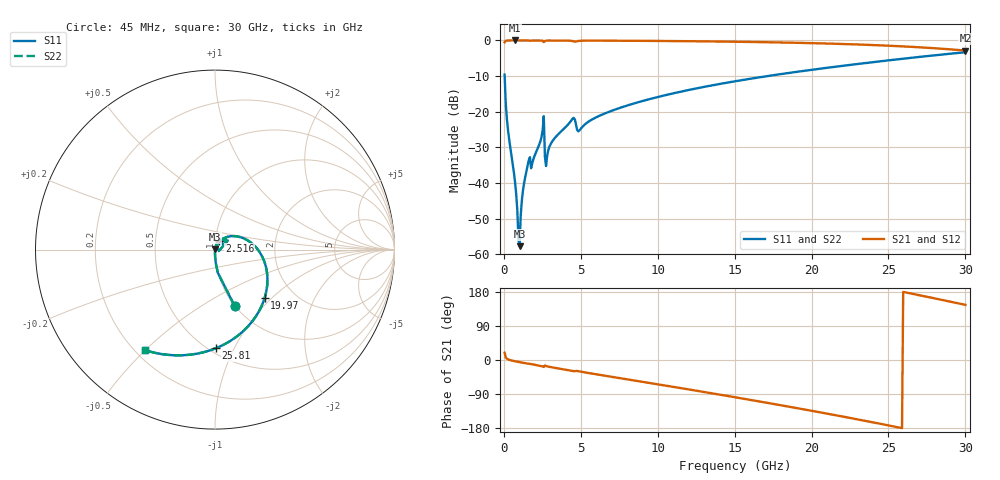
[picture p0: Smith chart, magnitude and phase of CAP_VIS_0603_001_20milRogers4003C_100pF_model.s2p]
! S-parameter model data by Modelithics Inc.  support@modelithics.com  813-866-6335  Tampa FL USA
! S-Parameter data specifications:
! Substrate: 20-mil Rogers 4003C, substrate thickness, H=0.508mm, Dielectric constant, Er=3.75
! PCB Mounting Pad Footprint: Pad width, PadW=0.90mm , Pad length, PadL=1.00mm , Pad gap, PadG (edge-to-edge)=1.00mm , Reference planes=3.0mm apart
! Created Wed Nov 18 13:31:23 2015
# hz S ma R 50
! 2 Port Network Data from SP1.SP block
! freq  magS11  angS11  magS21  angS21  magS12  angS12  magS22  angS22
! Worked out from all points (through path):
!   401 points, 45 MHz to 30 GHz, reference 50 ohm
!   highest |S21| = -0.01 dB at 719 MHz (marker M1); lowest = -2.8 dB at 30 GHz (marker M2)
!   group delay of S21, straight-line fit = 19.8 ps
!   lowest |S11| = -57.7 dB at 1.019 GHz (marker M3), VSWR 1.00, Z = 50.1 + j0.0984 ohm
!   |S11| at or under -10 dB: 48.8 MHz to 17.14 GHz (17.09 GHz wide, 199 % of centre)
!   |S22| runs from -57.7 to -3.3 dB; largest |S21 - S12| = 0
!   S11 on the Smith chart (normalised r, x): 45 MHz: 1.00, -0.70; 2.516 GHz: 1.04, +0.10; 19.97 GHz: 1.43, -0.90; 25.81 GHz: 0.54, -0.85; 30 GHz: 0.24, -0.50
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4.5e7  0.3317 -70.8  0.9432 19.1  0.9432 19.1  0.3317 -70.8
2.696625e8  0.0544 -87.9  0.9981 1.6  0.9981 1.6  0.0544 -87.9
7.189875e8  0.01049 -89.9  0.9993 -3.4  0.9993 -3.4  0.01049 -89.9
8.687625e8  0.004233 -85.2  0.9992 -4.5  0.9992 -4.5  0.004233 -85.2
1.018538e9  0.001298 49.2  0.9992 -5.7  0.9992 -5.7  0.001298 49.2
1.093425e9  0.003527 71.0  0.9991 -6.2  0.9991 -6.2  0.003527 71.0
1.318088e9  0.01015 77.0  0.9989 -7.8  0.9989 -7.8  0.01015 77.0
1.54275e9  0.01739 75.4  0.9982 -9.5  0.9982 -9.5  0.01739 75.4
1.917188e9  0.02161 73.6  0.9979 -11.8  0.9979 -11.8  0.02161 73.6
2.4414e9  0.0439 69.4  0.9953 -15.9  0.9953 -15.9  0.0439 69.4
2.516288e9  0.05505 64.4  0.99 -17.0  0.99 -17.0  0.05505 64.4
2.815838e9  0.02457 65.4  0.9962 -16.9  0.9962 -16.9  0.02457 65.4
3.190275e9  0.03969 67.7  0.9972 -19.8  0.9972 -19.8  0.03969 67.7
4.388475e9  0.0758 54.1  0.987 -28.4  0.987 -28.4  0.0758 54.1
5.062462e9  0.05997 52.2  0.9909 -31.2  0.9909 -31.2  0.05997 52.2
1.007992e10  0.1623 24.5  0.9835 -64.6  0.9835 -64.6  0.1623 24.5
1.50225e10  0.2673 -8.9  0.9593 -98.2  0.9593 -98.2  0.2673 -8.9
1.996508e10  0.386 -44.2  0.917 -133.7  0.917 -133.7  0.386 -44.2
2.003996e10  0.3879 -44.8  0.9162 -134.3  0.9162 -134.3  0.3879 -44.8
2.505742e10  0.5271 -83.5  0.8426 -173.1  0.8426 -173.1  0.5271 -83.5
2.58063e10  0.5498 -89.6  0.8279 -179.1  0.8279 -179.1  0.5498 -89.6
3e10  0.683 -124.9  0.721 145.5  0.721 145.5  0.683 -124.9
